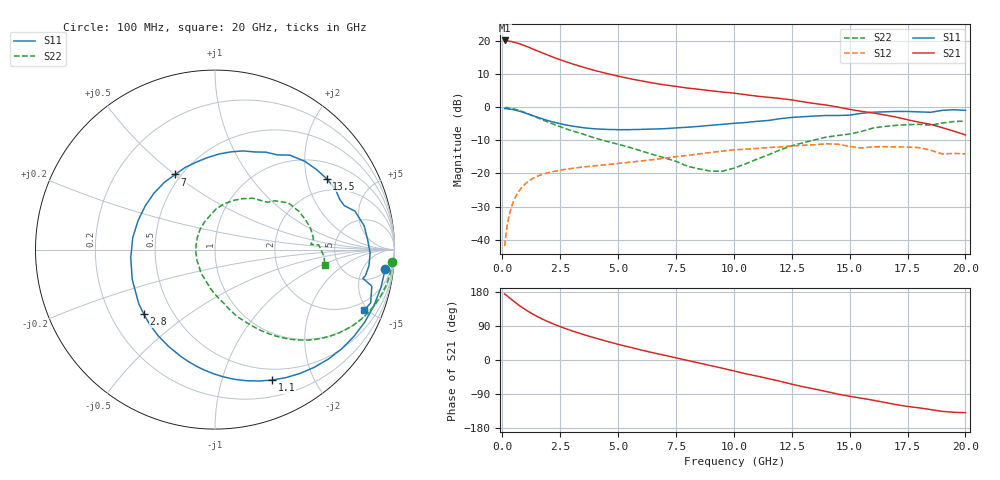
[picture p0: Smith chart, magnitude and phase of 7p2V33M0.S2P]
! Infineon Technologies  Discrete & RF Semiconductors
! bfp620
! VCE =  2.3 V,  IC =  3.0 mA
! Common Emitter S-Parameters:  Sep 2002
# GHz  S  MA  R  50
!  f  S11  S21  S12  S22
! GHz  MAG  ANG  MAG  ANG  MAG  ANG  MAG  ANG
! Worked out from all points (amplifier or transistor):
!   59 points, 100 MHz to 20 GHz, reference 50 ohm
!   highest |S21| = 20.2 dB at 100 MHz (marker M1)
!   |S21| within 3 dB of that: start of sweep to 1.463 GHz
!   unconditionally stable (mu >= 1): 5.319 GHz to 12.33 GHz; 14.34 GHz to 15.55 GHz; 17.46 GHz to end of sweep
!   at 1 GHz: K = 0.22, MSG = 20.8 dB, |S12| = -23.1 dB
!   at 5.5 GHz: K = 1.02, MAG = 11.8 dB, |S12| = -16.6 dB
!   at 20 GHz: K = 1.31, MAG = -0.5 dB, |S12| = -14.1 dB
!   S11 on the Smith chart (normalised r, x): 100 MHz: 6, -15; 1.1 GHz: 0.37, -1.47; 2.8 GHz: 0.34, -0.35; 7 GHz: 0.46, +0.50; 13.5 GHz: 1.52, +2.64; 20 GHz: 1.36, -4.72
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0.1  0.9551 -6.4  10.18 174.3  0.008 76.4  0.9907 -3.9
0.3  0.9391 -19.3  9.916 164.6  0.0238 77.6  0.975 -11.5
0.5  0.9131 -31.9  9.581 154.7  0.0391 71.6  0.9437 -18.8
0.6  0.8966 -38.0  9.381 150.0  0.0462 68.3  0.9236 -22.3
0.8  0.8581 -49.8  8.922 141.1  0.0591 61.9  0.8772 -28.8
1.1  0.7937 -66.3  8.139 129.0  0.075 53.2  0.7997 -37.2
1.5  0.7106 -86.2  7.12 115.0  0.0905 43.8  0.6984 -46.2
1.9  0.6399 -103.7  6.254 103.2  0.1011 36.7  0.6116 -53.1
2.4  0.5747 -123.5  5.358 90.4  0.1106 30.0  0.5236 -60.0
2.8  0.5357 -137.7  4.799 81.5  0.1165 25.7  0.4658 -64.6
3.5  0.4903 -160.2  4.018 67.2  0.1255 19.7  0.392 -71.8
4  0.4715 -174.6  3.583 58.2  0.1305 16.1  0.343 -76.4
5  0.4582 159.2  2.946 41.4  0.1418 10.7  0.2764 -84.8
6  0.4632 137.1  2.502 26.4  0.1546 5.7  0.2194 -96.3
7  0.4741 117.9  2.177 12.6  0.1698 0.7  0.1723 -109.7
9  0.5333 87.5  1.775 -14.9  0.2076 -12.8  0.1083 -170.3
10.5  0.5876 67.8  1.548 -36.2  0.2329 -26.4  0.1396 126.7
12  0.6717 51.6  1.356 -56.2  0.2516 -38.6  0.2274 88.2
13.5  0.7371 32.5  1.135 -76.8  0.2725 -53.3  0.3223 61.7
15  0.7607 18.8  0.929 -95.7  0.2567 -72.7  0.3938 42.1
17  0.8644 -1.2  0.711 -117.6  0.252 -84.4  0.5315 18.1
20  0.8973 -22.2  0.382 -138.9  0.1983 -102.3  0.6181 -7.8
